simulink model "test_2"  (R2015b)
settings: Solver=VariableStepAuto  StartTime=0.0  StopTime=200.0  RelTol=1e-3
undefined symbols (not defined in the file or in its folder): fir1
libraries: simulink x1, dspstat3 x1

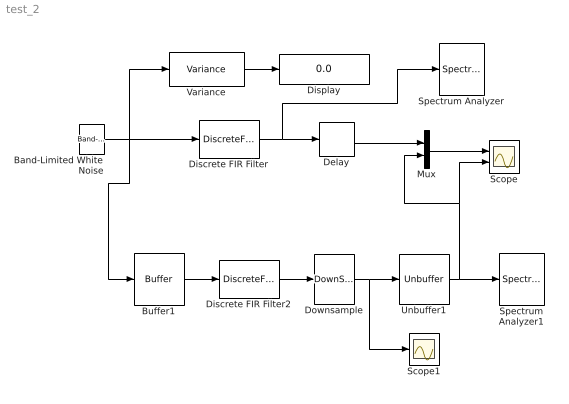
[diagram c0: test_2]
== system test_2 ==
  Band-Limited White Noise : simulink/Sources/Band-Limited White Noise  Cov=[0.01]  Ts=0.01  seed=[23341]
  Buffer1 : Buffer  N=2048  TreatMby1Signals=One channel  OutputFrames=off
  Delay : Delay  DelayLength=5*2048
  Discrete FIR Filter : DiscreteFir  Coefficients=fir1(256, 0.2);
  Discrete FIR Filter2 : DiscreteFir  Coefficients=fir1(256, 0.2);  InputProcessing=Columns as channels (frame based)
  Display : Display
  Downsample : DownSample  N=4  RateOptions=Allow multirate processing
  Mux : Mux  Inputs=2
  Scope : Scope  NumInputPorts=2
  Scope1 : Scope
  Spectrum Analyzer : SpectrumAnalyzer
  Spectrum Analyzer1 : SpectrumAnalyzer
  Unbuffer1 : Unbuffer  SampleBasedProcessing=Same as frame based
  Variance : dspstat3/Variance  run=on  reset_popup=None  directionMode=Each column  dimension=1  roiEnable=off  roiType=Rectangles  roiPortion=Entire ROI  roiOutput=Individual statistics for each ROI  roiFlag=off  roundingMode=Floor  overflowMode=off
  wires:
  Band-Limited White Noise/1 -> Variance/1, Discrete FIR Filter/1, Buffer1/1
  Mux/1 -> Scope/1
  Variance/1 -> Display/1
  Buffer1/1 -> Discrete FIR Filter2/1
  Discrete FIR Filter2/1 -> Downsample/1
  Downsample/1 -> Scope1/1, Unbuffer1/1
  Discrete FIR Filter/1 -> Delay/1, Spectrum Analyzer/1
  Delay/1 -> Mux/1
  Unbuffer1/1 -> Mux/2, Scope/2, Spectrum Analyzer1/1
